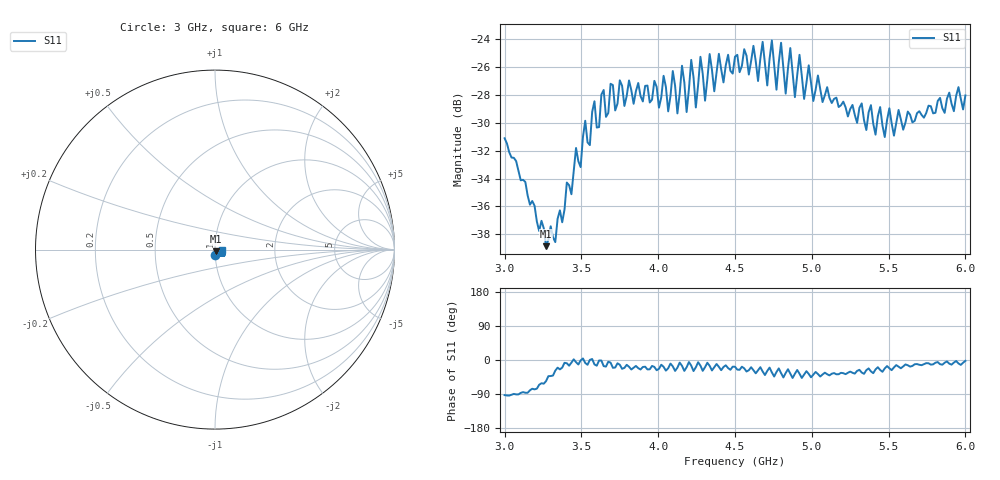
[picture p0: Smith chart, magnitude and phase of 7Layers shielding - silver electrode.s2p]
!  03/07/2025  16:44:39
! Ref Plane: 0.000 mm
# MHZ S MA R  50
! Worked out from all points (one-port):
!   201 points, 3 GHz to 6 GHz, reference 50 ohm
!   lowest |S11| = -38.8 dB at 3.27 GHz (marker M1), VSWR 1.02, Z = 50.6 - j0.955 ohm
!   |S11| at or under -10 dB: start of sweep to end of sweep
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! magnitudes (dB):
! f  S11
! 3 GHz  -31.1
! 3.27 GHz  -38.8
! 3.375 GHz  -37.1
! 3.525 GHz  -29.9
! 3.555 GHz  -31.6
! 3.585 GHz  -28.5
! 3.615 GHz  -30.3
! 3.75 GHz  -27.0
! 4.005 GHz  -28.9
! 4.035 GHz  -26.6
! 4.065 GHz  -29.2
! 4.095 GHz  -26.3
! 4.125 GHz  -29.3
! 4.155 GHz  -25.9
! 4.185 GHz  -29.2
! 4.215 GHz  -25.5
! 4.245 GHz  -28.9
! 4.275 GHz  -25.3
! 4.305 GHz  -28.4
! 4.335 GHz  -25.1
! 4.365 GHz  -27.7
! 4.395 GHz  -25.1
! 4.425 GHz  -27.1
! 4.5 GHz  -25.3
! 4.875 GHz  -26.4
! 5.25 GHz  -29.0
! 5.625 GHz  -29.2
! 6 GHz  -28.0
